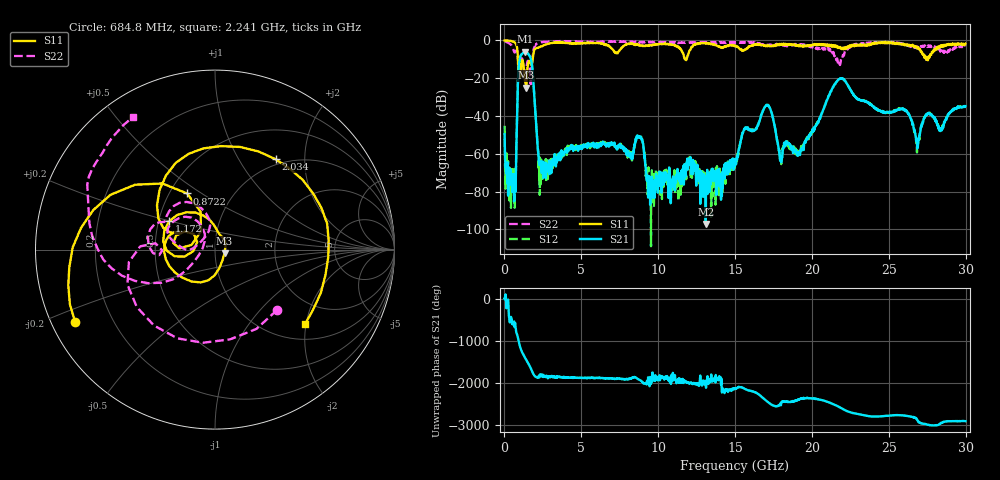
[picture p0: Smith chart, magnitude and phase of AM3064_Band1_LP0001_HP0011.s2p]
# Hz S DB R 50.0
!freq dBS11 angS11 dBS21 angS21 dBS12 angS12 dBS22 angS22
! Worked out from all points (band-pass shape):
!   1600 points, 10 MHz to 29.98 GHz, reference 50 ohm
!   highest |S21| = -5.95 dB at 1.36 GHz (marker M1); lowest = -97.2 dB at 13.09 GHz (marker M2)
!   |S21| within 3 dB of the highest: 1.023 GHz to 1.681 GHz (657.9 MHz wide, 48.7 % of centre)
!   lowest |S11| = -24.9 dB at 1.416 GHz (marker M3), VSWR 1.12, Z = 55.6 - j2.18 ohm
!   |S11| at or under -10 dB: 876.5 MHz to 1.829 GHz (952.9 MHz wide, 70.4 % of centre); 11.74 GHz to 11.84 GHz (100.7 MHz wide, 0.854 % of centre); 27.5109 GHz to 27.55298 GHz (42.08 MHz wide, 0.153 % of centre)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
!   |S22| runs from -23.2 to -0.2 dB; largest |S21 - S12| = 0.0055
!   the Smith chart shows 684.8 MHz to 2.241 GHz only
!   S11 on the Smith chart (normalised r, x): 684.8 MHz: 0.07, -0.24; 872.2 MHz: 0.61, +0.44; 1.172 GHz: 0.57, +0.20; 2.034 GHz: 0.91, +1.46; 2.241 GHz: 1.37, -1.98
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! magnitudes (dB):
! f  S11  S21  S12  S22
! 10 MHz  -0.1  -49.8  -45.2  -0.2
! 403.6 MHz  -0.3  -70.3  -68.8  -2.2
! 684.8 MHz  -1.1  -70.9  -71.9  -6.3
! 872.2 MHz  -9.1  -23.1  -23.1  -9.5
! 1.172 GHz  -10.4  -6.9  -6.8  -10.2
! 1.36 GHz  -22.1  -5.9  -6.0  -18.2
! 1.416 GHz  -24.9  -6.1  -6.1  -15.2
! 2.034 GHz  -4.3  -41.0  -40.9  -2.2
! 2.241 GHz  -3.7  -64.5  -64.4  -1.2
! 5.015 GHz  -1.4  -56.0  -56.2  -0.7
! 8.745 GHz  -2.7  -51.5  -51.0  -1.2
! 9.382 GHz  -2.8  -80.1  -72.4  -0.7
! 10 GHz  -2.0  -73.1  -72.4  -0.9
! 13.09 GHz  -1.5  -97.2  -77.6  -0.9
! 15 GHz  -3.0  -65.7  -64.6  -1.2
! 17.05 GHz  -2.9  -34.3  -34.3  -2.7
! 17.97 GHz  -2.4  -62.0  -60.8  -2.1
! 19.99 GHz  -2.7  -48.4  -48.3  -3.4
! 21.83 GHz  -3.8  -20.4  -20.3  -13.0
! 25 GHz  -1.0  -38.2  -38.1  -1.1
! 26.85 GHz  -4.2  -57.2  -55.3  -3.2
! 29.98 GHz  -1.8  -34.8  -35.3  -3.2
